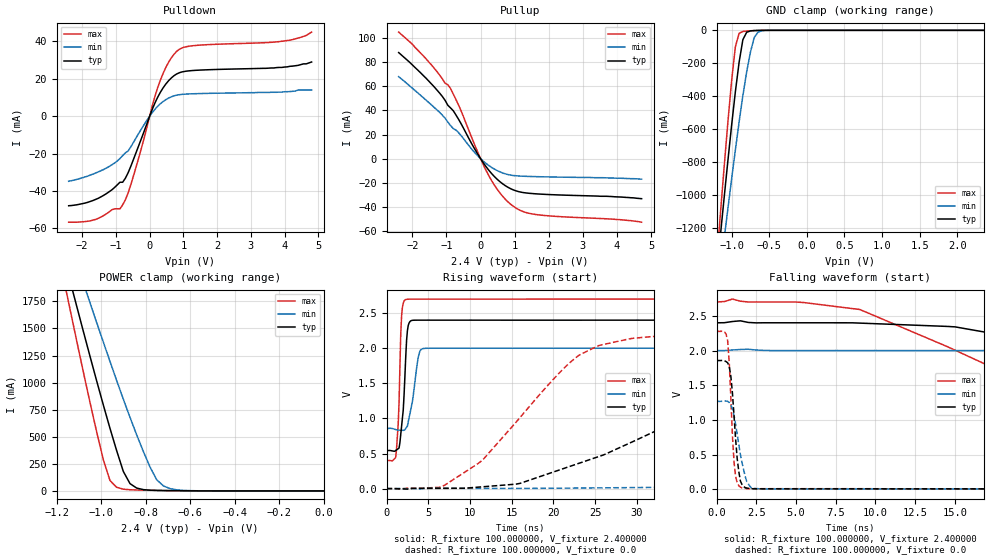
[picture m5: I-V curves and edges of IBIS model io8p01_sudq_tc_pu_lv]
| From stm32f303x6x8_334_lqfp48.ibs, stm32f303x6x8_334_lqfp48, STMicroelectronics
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|   Model io8p01_sudq_tc_pu_lv
[Model]  io8p01_sudq_tc_pu_lv
Model_type I/O
Polarity   Non-Inverting
Enable   Active-Low
Vinl =   0.720000V
Vinh =   1.680000V
Vmeas =  1.200000V
Cref =   50.000000pF
Rref =   100.000000M
Vref =   0.0V
C_comp   1.378000pF   1.292700pF   1.486400pF
[Temperature Range]   25.000000   0.125000k   -40.000000
[Pullup Reference]   2.400000V   2.000000V   2.700000V
[Pulldown Reference]   0.0V   0.0V   0.0V
[POWER Clamp Reference]   2.400000V   2.000000V   2.700000V
[GND Clamp Reference]   0.0V   0.0V   0.0V
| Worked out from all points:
|   slope of the pulldown table from 0 to 0.36 V, typ, clamps not added: 25.7 ohm
|   slope of the pullup table from 0 to 0.36 V, typ, clamps not added: 26.8 ohm
|   GND clamp passes 1 mA (typ) near -0.67 V on its own axis
|   POWER clamp passes 1 mA (typ) near -0.60 V on its own axis
|   rising waveform, R_fixture 100.000000, V_fixture 2.400000: 20-80 % time 540ps typ, 838ps min, 354ps max; typ from 0.543 V to 2.4 V
|   rising waveform, R_fixture 100.000000, V_fixture 0.0: 20-80 % time 22.5ns typ, 62.6ns min, 10.4ns max; typ from 0.001 V to 1.86 V
|   falling waveform, R_fixture 100.000000, V_fixture 2.400000: 20-80 % time 28.7ns typ, 66.4ns min, 14.8ns max; typ from 2.4 V to 0.543 V
|   falling waveform, R_fixture 100.000000, V_fixture 0.0: 20-80 % time 377ps typ, 594ps min, 284ps max; typ from 1.86 V to 0.001 V
[Pulldown]
|Voltage   I(typ)   I(min)   I(max)
-2.4V     -47.9mA    -34.8mA    -56.7mA
-1.6V     -44.5mA    -30.4mA    -55.2mA
-880mV    -35.33mA   -22.63mA   -49.55mA
-800mV    -35.33mA   -21.13mA   -47.42mA
-640mV    -30.33mA   -18.65mA   -41.16mA
-480mV    -23.12mA   -14mA      -31.94mA
240mV     10.22mA    5.339mA    15.38mA
480mV     17.22mA    8.864mA    26.1mA
800mV     22.59mA    11.27mA    34.68mA
1.28V     24.44mA    12mA       37.7mA
4.16V     26.7mA     13.2mA     40.7mA
4.8V      29mA       14mA       45mA
[Pullup]
|Voltage   I(typ)   I(min)   I(max)
-2.4V     88mA       68mA       105mA
-2V       77.8mA     58.5mA     95mA
-1.36V    59.6mA     42.5mA     75.1mA
-880mV    42.12mA    27.44mA    58.22mA
-560mV    28.45mA    18.75mA    39mA
-160mV    7.44mA     4.66mA     10.64mA
160mV     -6.607mA   -3.947mA   -9.704mA
480mV     -16.91mA   -9.806mA   -25.1mA
880mV     -24.89mA   -13.63mA   -37.75mA
1.2V      -27.87mA   -14.5mA    -43.37mA
1.6V      -29.13mA   -14.89mA   -46.24mA
4.72V     -33.2mA    -17mA      -52.7mA
[GND_clamp]
|Voltage   I(typ)   I(min)   I(max)
-2.4V     -7.358A    -6.372A    -8.78A
-1.2V     -1.489A    -1.65A     -1.416A
-1.15V    -1.254A    -1.461A    -1.124A
-1.1V     -1.024A    -1.273A    -838.2mA
-1.05V    -797.6mA   -1.088A    -563.1mA
-950mV    -374.6mA   -728.7mA   -100.8mA
-900mV    -194.3mA   -557.9mA   -18.01mA
-850mV    -56.94mA   -397.4mA   -7.08mA
-750mV    -3.582mA   -133.8mA   -2.771mA
-700mV    -1.516mA   -44.7mA    -1.516mA
-600mV    -235.4uA   -2.939mA   -209.5uA
2.35V     0A         0A         0A
[POWER_clamp]
|Voltage   I(typ)   I(min)   I(max)
-2.4V     9.979A     9.967A     9.901A
-1.17V    2.182A     2.481A     1.978A
-1.14V    1.945A     2.294A     1.683A
-1.11V    1.71A      2.108A     1.391A
-1.08V    1.476A     1.923A     1.102A
-1.05V    1.245A     1.739A     819.9mA
-960mV    578.3mA    1.196A     96.08mA
-900mV    179.5mA    846.7mA    16.05mA
-870mV    67.19mA    678.8mA    10.83mA
-780mV    6.763mA    219.9mA    5.868mA
-720mV    3.368mA    46.35mA    3.823mA
0V        0A         0A         0A
[Ramp]
| variable   typ   min   max
dV/dt_r  1.11273/22.42683n   0.75702/62.77895n   1.36520/10.35560n
dV/dt_f  1.11418/28.66195n   0.68660/66.52286n   1.37899/14.74510n
R_load = 100.000000
[Rising Waveform]
R_fixture= 100.000000
V_fixture= 2.400000
V_fixture_min= 2.000000
V_fixture_max= 2.700000
|time   V(typ)   V(min)   V(max)
0s        543.1mV    857mV      401.7mV
1.101ns   543mV      841.3mV    444.3mV
1.401ns   569.8mV    834.3mV    922.7mV
1.802ns   884.9mV    831.3mV    2.455V
2.002ns   1.117V     829.8mV    2.641V
2.302ns   1.876V     856.5mV    2.693V
2.703ns   2.359V     1.008V     2.699V
3.804ns   2.4V       1.871V     2.699V
4.404ns   2.4V       1.995V     2.699V
49.85ns   2.4V       2V         2.7V
[Rising Waveform]
R_fixture= 100.000000
V_fixture= 0.0
V_fixture_min= 0.0
V_fixture_max= 0.0
|time   V(typ)   V(min)   V(max)
0s        956.5uV    1.197mV    860.5uV
6.507ns   5.37mV     4.195mV    20.52mV
11.01ns   21.95mV    4.215mV    360.7mV
16.02ns   75.83mV    4.316mV    1.016V
23.52ns   379.9mV    9.446mV    1.928V
37.04ns   1.079V     61.58mV    2.22V
52.55ns   1.658V     194.2mV    2.266V
75.58ns   1.814V     478.5mV    2.276V
139.1ns   1.855V     1.133V     2.276V
249.2ns   1.856V     1.267V     2.276V
[Falling Waveform]
R_fixture= 100.000000
V_fixture= 2.400000
V_fixture_min= 2.000000
V_fixture_max= 2.700000
|time   V(typ)   V(min)   V(max)
0s        2.4V       2V         2.7V
9.009ns   2.396V     2V         2.592V
15.02ns   2.341V     2V         2.005V
28.03ns   1.809V     1.956V     817.7mV
33.53ns   1.559V     1.925V     582.4mV
40.04ns   1.293V     1.873V     493.7mV
55.56ns   817.5mV    1.669V     429.5mV
73.57ns   630mV      1.448V     409mV
126.1ns   551.7mV    1.018V     401.6mV
249.2ns   543.1mV    857mV      401.7mV
[Falling Waveform]
R_fixture= 100.000000
V_fixture= 0.0
V_fixture_min= 0.0
V_fixture_max= 0.0
|time   V(typ)   V(min)   V(max)
0s        1.856V     1.267V     2.276V
700.7ps   1.824V     1.266V     2.141V
900.9ps   1.631V     1.21V      1.321V
1.101ns   1.061V     1.064V     393.1mV
1.201ns   722.1mV    935.5mV    184.1mV
1.401ns   255.7mV    643.5mV    50.88mV
1.702ns   39.42mV    285.7mV    13.58mV
2.202ns   8.094mV    16.68mV    7.773mV
2.903ns   5.642mV    4.558mV    7.628mV
49.85ns   956.5uV    1.197mV    860.5uV
